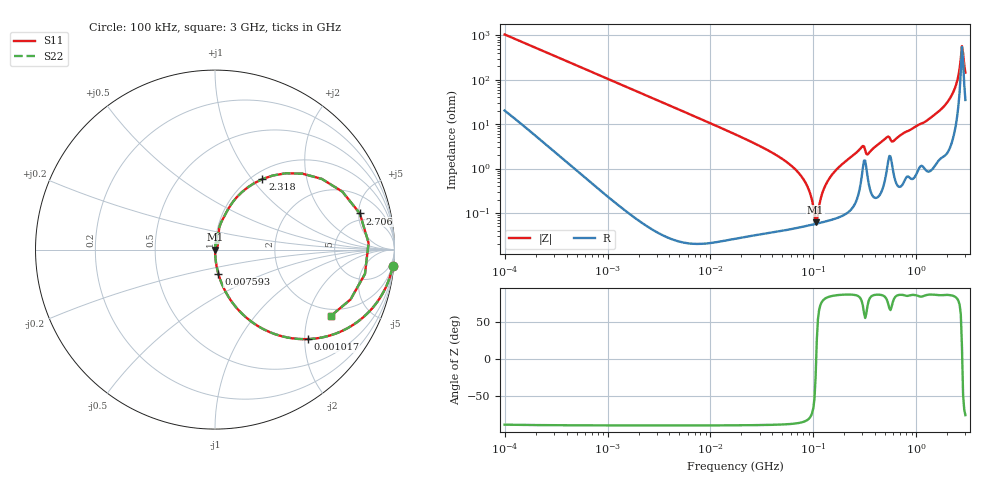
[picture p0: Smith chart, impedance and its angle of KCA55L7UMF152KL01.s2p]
!Murata Part Number: KCA55L7UMF152KL01
!These Parameters are Measured in Series Mode Connection
!Data Generated on Jan 08, 2026
!  o--ll--o
!Port1  Port2
!  o------o
!Operation Temp=25[degC], DC Bias Voltage=0[V]
!Freq. Start=100[kHz] Stop=3[GHz] 401[Steps]
# Hz S RI R 50
!Freq.(Hz) S11(Real) S11(Imag) S21(Real) S21(Imag) S12(Real) S12(Imag) S22(Real) S22(Imag)
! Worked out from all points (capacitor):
!   401 points, 100 kHz to 3 GHz, reference 50 ohm
!   read as one part in series: C = 1.51 nF near 105.3 kHz
!   lowest |Z| = 61.7 mohm at 105.2 MHz (marker M1)
!   series resonance near 106.5 MHz, so ESL is about 1.5 nH
!   S11 on the Smith chart (normalised r, x): 100 kHz: 1, -21; 1.017 MHz: 1.00, -2.08; 7.593 MHz: 1.00, -0.28; 2.318 GHz: 1.11, +1.13; 2.706 GHz: 3.96, +5.17; 3 GHz: 1.70, -2.81
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100000  0.9892 -0.0941  0.0108 0.0941  0.0108 0.0941  0.9892 -0.0941
562235  0.778 -0.4137  0.222 0.4137  0.222 0.4137  0.778 -0.4137
1017073  0.5184 -0.4986  0.4816 0.4986  0.4816 0.4986  0.5184 -0.4986
3161081  0.1004 -0.3  0.8996 0.3  0.8996 0.3  0.1004 -0.3
7592607  0.0189 -0.1356  0.9811 0.1356  0.9811 0.1356  0.0189 -0.1356
1.77727e7  0.00357 -0.0574  0.9964 0.0574  0.9964 0.0574  0.00357 -0.0574
6.283488e7  0.000555 -0.0109  0.9994 0.0109  0.9994 0.0109  0.000555 -0.0109
8.342988e7  0.000524 -0.00487  0.9995 0.00487  0.9995 0.00487  0.000524 -0.00487
9.738194e7  0.000545 -0.00178  0.9995 0.00178  0.9995 0.00178  0.000545 -0.00178
1.0521e8  0.000565 -0.000248  0.9994 0.000248  0.9994 0.000248  0.000565 -0.000248
1.107752e8  0.000581 0.00077  0.9994 -0.00077  0.9994 -0.00077  0.000581 0.00077
1.293002e8  0.000649 0.00386  0.9994 -0.00386  0.9994 -0.00386  0.000649 0.00386
1.673121e8  0.000843 0.00936  0.9992 -0.00936  0.9992 -0.00936  0.000843 0.00936
2.94964e8  0.00737 0.0293  0.9926 -0.0293  0.9926 -0.0293  0.00737 0.0293
3.442911e8  0.00509 0.0212  0.9949 -0.0212  0.9949 -0.0212  0.00509 0.0212
5.475153e8  0.0209 0.0451  0.9791 -0.0451  0.9791 -0.0451  0.0209 0.0451
1.281618e9  0.0229 0.1186  0.9771 -0.1186  0.9771 -0.1186  0.0229 0.1186
1.935725e9  0.0888 0.2504  0.9112 -0.2504  0.9112 -0.2504  0.0888 0.2504
2.318426e9  0.2638 0.3928  0.7362 -0.3928  0.7362 -0.3928  0.2638 0.3928
2.504792e9  0.4869 0.4231  0.5131 -0.4231  0.5131 -0.4231  0.4869 0.4231
2.706139e9  0.8068 0.2014  0.1932 -0.2014  0.1932 -0.2014  0.8068 0.2014
3e9  0.645 -0.3699  0.355 0.3699  0.355 0.3699  0.645 -0.3699
